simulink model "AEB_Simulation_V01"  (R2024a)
settings: Solver=ode23tb  StartTime=0.0  StopTime=inf  RelTol=2e-1
PreLoadFcn:
  | helperCreateDetectorBus;
model workspace (MAT data in the model file):
  EngPwr = 352122.842504
  EngWc = 4.047
  Tdiff = 849
  Tlim = 1000
  VEH : object (value not decoded)
undefined symbols (not defined in the file or in its folder): automotive_project_windows, blkdiag, C, car, D, Female, MATLAB, Performance, R2024a, Row, shared, sim3d_projects, Sim3dSensor, toolbox, UE, vector, VehicleSimulation, WindowsNoEditor
libraries: simulink x7, sim3dautolib x4, vehdynlibtirecommon x4, autolibutils x4, sharedtransform x2, sim3dcameralib x1, sim3dphyssensorlib x1, sim3dlib x1, motalgorithmslib x1, vehdynlibtire x1, vehdynlibsteering x1, autolibshared x1
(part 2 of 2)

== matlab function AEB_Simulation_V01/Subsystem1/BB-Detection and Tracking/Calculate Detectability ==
function detectableTracksInput = CalculateDetectability(allTracks, positionIndices)
% This function calculates the probability of detection for each track. The
% helperCalcDetectability function is used to compute the probability after
% extracting the tracks from the bus.
tracks = allTracks.Tracks(1:allTracks.NumTracks);
detectableTracksInput = helperCalcDetectability(tracks, positionIndices);
end

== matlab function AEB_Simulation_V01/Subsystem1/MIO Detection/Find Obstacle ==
function [x,vx,mioTrack] = findObstacle(confirmedTracks, curvature, positionSelector)
% This function finds the lead car: a car in front of the ego car that
% satisfies all the criteria below:
% * Within the ego car's lane.
% * In front of the ego car.
% * Closest to the ego car.

% Important notes:
% 1. If you change state definition, change the following:
%       State = [x;vx;y;vy;z;vz] (3D constant velocity)
numStates = 6;

% 2. The lane is defined using a parabolic model, where y=ax^2+bx+c. a is
%    equal to half the road curvature, b=0, and c is the offset of the lane
%    boundaries relative to the ego car. Overall lane width is assumed to
%    be 3.6m, typical highway lane width.
laneWidth = 3.6;

% 3. The ego car is assumed to be traveling in the middle of its lane, with
%    1.8m on each side of it. So, c=+1.8m for the left lane boundary and
%    -1.8m for the right lane boundary.
halfLaneWidth = laneWidth/2;

% Initialize outputs and parameters
maxX = cast(1000, 'like', confirmedTracks.Tracks(1).State);  % Far enough forward so that no track is expected to exceed this distance
trackID = 0;

for i = 1:confirmedTracks.NumTracks
    % position = positionSelector * confirmedTracks.Tracks(i).State;
    % x = position(1); % Longitudinal position of the track relative to ego
    % y = position(2); % Lateral position of the track relative to ego

    x = 0;
    y = 0;
    
    if x < maxX && x > 0 % No point checking otherwise
        yleftLane  = polyval([curvature/2, 0,  halfLaneWidth],x); % Half a lane to the left
        yrightLane = polyval([curvature/2, 0, -halfLaneWidth],x); % Half a lane to the right
        
        % Find a new lead car
        if (yrightLane <= y) && (y <= yleftLane)
            maxX = x;
            trackID = i;
        end
    end
end

if trackID>0
    mioState = confirmedTracks.Tracks(trackID).State;
else
    mioState = inf(numStates,1,'like',confirmedTracks.Tracks(1).State);
end

% Output:
x = mioState(1);    % Longitudinal position of the lead car
vx = mioState(2);   % Longitudinal velocity of the lead car
mioTrack = confirmedTracks.Tracks(1).State %trackID; % Index of the most important track

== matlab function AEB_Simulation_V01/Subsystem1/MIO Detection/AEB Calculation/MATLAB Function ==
function AEB  = fcn(x_obj, th_AEB)

AEB = 0;

if (x_obj < th_AEB(1))
    AEB = 1.0;
end

if (x_obj < th_AEB(2))
    AEB = 2.0;
end

if (x_obj < th_AEB(3))
    AEB = 3.0;
end
